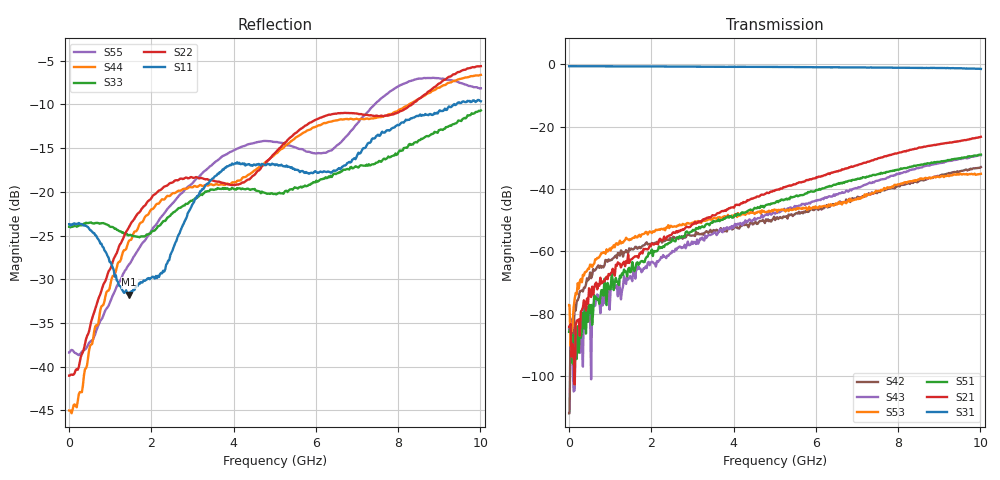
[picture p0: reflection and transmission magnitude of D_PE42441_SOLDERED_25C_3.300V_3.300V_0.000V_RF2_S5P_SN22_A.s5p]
! Device ID: PE42441
! Serial: 22
! Insertion: A
! Temp: 25C
! VDD: 3.300
! Control_Hi: 100.000
! Control_Lo: 0.000
! Logic State: RF2
! Port 1: RFC
! Port 2: RF1
! Port 3: RF2
! Port 4: RF3
! Port 5: RF4
! V1 = 3.30
! V2 = 0.00
! V3 = 0.00
! V4 = 0.00
! IDD: 1.081577e-04
! 1 Hz data is simulated
#  Hz  S  RI  R  50
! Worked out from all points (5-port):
!   402 points, 1 Hz to 10.01 GHz, reference 50 ohm
!   strongest paths, dB at 1 Hz, 2.485 GHz, 5.01 GHz, 7.51 GHz, 10.01 GHz:
!     S31: -0.7, -0.8, -0.9, -1.1, -1.5
!     S21: -84.2, -54.7, -40.3, -30.1, -23.3
!     S51: -85.7, -56.9, -44.5, -35.3, -29.0
!     S53: -77.1, -51.8, -46.7, -40.7, -35.1
!     S43: -84.7, -60.6, -47.9, -37.3, -29.2
!     S42: -111.8, -56.2, -49.9, -40.9, -33.0
!   lowest |S11| = -31.7 dB at 1.46 GHz (marker M1), VSWR 1.05, Z = 49.7 - j2.56 ohm
!   |S11| at or under -10 dB: start of sweep to 9.353 GHz; 9.367 GHz to 9.416 GHz (49.36 MHz wide, 0.526 % of centre)
